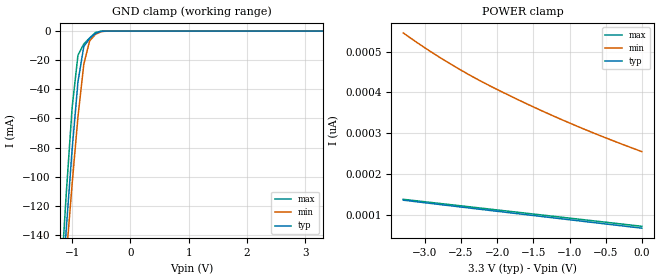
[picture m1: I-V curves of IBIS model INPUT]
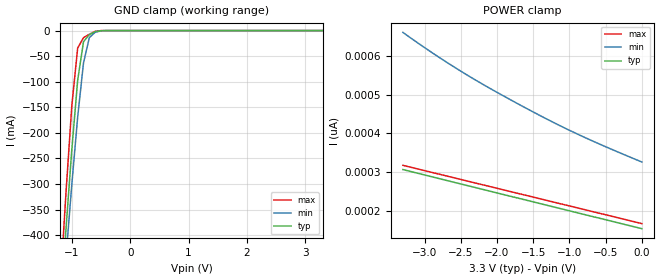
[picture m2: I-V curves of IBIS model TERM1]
|   PERICOM SEMICONDUCTOR CORP
|   IBIS Model of PI3C32X245
|   Product Family: 3C
|   BQSOP (B) Package
[IBIS Ver] 3.2
[Comment char] |_char
[File Name] pi3c32x245_b_33v.ibs
[File Rev] 2.0
[Source] File originated at Pericom Semiconductor Corp.
[Date] 03/15/18
[Disclaimer] (C) Copyright PERICOM Semiconductor Corporation
   All rights reserved
  Pericom Semiconductor Corporation hereby grants the user of
  this IBIS model a non-exclusive, nontransferable license to
  use this IBIS model under the following terms.
  This IBIS model is provided on an "AS IS" basis and Pericom
  makes absolutely no warranty with respect to the information
  contained herein. PERICOM DISCLAIMS AND CUSTOMER WAIVES ALL
  WARRANTIES, EXPRESSED OR IMPLIED, INCLUDING WARRANTIES OF
  MERCHANTABILITY OR FITNESS FOR A PARTICULAR PURPOSE. The
  entire risk as to quality and performance is with the customer.
  Accordingly, in no event shall the company be liable for any
  damages, whether in contract or tort, including any lost
  profits or other incidental, consequential, exemplary, or
  punitive damages arising out of the use or application of the
  IBIS model provided in this package. Further, Pericom reserves
  the right to make changes without notice to any product herein
  to improve reliability, function, or design. Pericom does not
  convey any license under patent rights or any other intellectual
  property rights, including those of third parties.
  The user is granted this license only to use the IBIS model
  and is not granted rights to sell, load, rent, lease or license
  the IBIS model in whole or in part, or in modified form to anyone
  other than user. User may modify the IBIS model to suit its specific
  application but rights to derivative works and such modifications
  shall belong to Pericom.
  Pericom is not obligated to provide maintenance or support
  for the licensed IBIS model.
  Contact Pericom at ATTN: APPLICATION ENGINEERING / IBIS MODELS
  2380 Bering Drive, San Jose, CA 95131
[Component] PI3C32X245
[Manufacturer] Pericom Semiconductor Corp.
[Package]
| Variable   typ   min   max
R_pkg   0.03818ohm   0.02666ohm   0.04970ohm
L_pkg   0.79246nH   0.73792nH   0.84700nH
C_pkg   0.19953pF   0.16164pF   0.23742pF
[Pin]  signal_name   model_name   R_pin   L_pin   C_pin
1   NC   NC   0.04970   0.84700nH   0.23742pF
2   A0   TERM1   0.04714   0.83488nH   0.22900pF
3   A1   TERM1   0.04458   0.82276nH   0.22058pF
4   A2   TERM1   0.04202   0.81064nH   0.21216pF
5   A3   TERM1   0.03946   0.79852nH   0.20374pF
6   A4   TERM1   0.03690   0.78640nH   0.19532pF
7   A5   TERM1   0.03434   0.77428nH   0.18690pF
8   A6   TERM1   0.03178   0.76216nH   0.17848pF
9   A7   TERM1   0.02922   0.75004nH   0.17006pF
10   GND   GND   0.02666   0.73792nH   0.16164pF
11   NC   NC   0.02666   0.73792nH   0.16164pF
12   A8   TERM1   0.02922   0.75004nH   0.17006pF
13   A9   TERM1   0.03178   0.76216nH   0.17848pF
14   A10   TERM1   0.03434   0.77428nH   0.18690pF
15   A11   TERM1   0.03690   0.78640nH   0.19532pF
16   A12   TERM1   0.03946   0.79852nH   0.20374pF
17   A13   TERM1   0.04202   0.81064nH   0.21216pF
18   A14   TERM1   0.04458   0.82276nH   0.22058pF
19   A15   TERM1   0.04714   0.83488nH   0.22900pF
20   GND   GND   0.04970   0.84700nH   0.23742pF
21   B15   TERM2   0.04970   0.84700nH   0.23742pF
22   B14   TERM2   0.04714   0.83488nH   0.22900pF
23   B13   TERM2   0.04458   0.82276nH   0.22058pF
24   B12   TERM2   0.04202   0.81064nH   0.21216pF
25   B11   TERM2   0.03946   0.79852nH   0.20374pF
26   B10   TERM2   0.03690   0.78640nH   0.19532pF
27   B9   TERM2   0.03434   0.77428nH   0.18690pF
28   B8   TERM2   0.03178   0.76216nH   0.17848pF
29   _BE2   INPUT   0.02922   0.75004nH   0.17006pF
30   VCC   POWER   0.02666   0.73792nH   0.16164pF
31   B7   TERM2   0.02666   0.73792nH   0.16164pF
32   B6   TERM2   0.02922   0.75004nH   0.17006pF
33   B5   TERM2   0.03178   0.76216nH   0.17848pF
34   B4   TERM2   0.03434   0.77428nH   0.18690pF
35   B3   TERM2   0.03690   0.78640nH   0.19532pF
36   B2   TERM2   0.03946   0.79852nH   0.20374pF
37   B1   TERM2   0.04202   0.81064nH   0.21216pF
38   B0   TERM2   0.04458   0.82276nH   0.22058pF
39   _BE1   INPUT   0.04714   0.83488nH   0.22900pF
40   VCC   POWER   0.04970   0.84700nH   0.23742pF
[Series Switch Groups]
On 1 /
Off 2 /
[Series Pin Mapping]   pin_2   model_name  function_table_group
2   38   SWITCH1   1
3   37   SWITCH1   1
4   36   SWITCH1   1
5   35   SWITCH1   1
6   34   SWITCH1   1
7   33   SWITCH1   1
8   32   SWITCH1   1
9   31   SWITCH1   1
12   28   SWITCH1   2
13   27   SWITCH1   2
14   26   SWITCH1   2
15   25   SWITCH1   2
16   24   SWITCH1   2
17   23   SWITCH1   2
18   22   SWITCH1   2
19   21   SWITCH1   2
|   Model SWITCH1
[Model] SWITCH1
Model_type Series_switch
| variable   typ   min   max
C_comp   10.000pF   9.800pF   10.200pF
[Voltage Range]   3.3000V   2.9700V   3.6300V
[GND Clamp Reference]   0.0000V   0.0000V   0.0000V
[POWER Clamp Reference]   3.3000V   2.9700V   3.6300V
[Temperature Range]   25   85   -40
[On]
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[OFF]
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| Models and submodels in the file (4): INPUT (Input), SWITCH1 (Series_switch), TERM1 (Terminator), TERM2 (Terminator)
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|   Model INPUT
[Model] INPUT
Model_type Input
Vinl = 800mV
Vinh = 2.0V
| variable   typ   min   max
C_comp   3.500pF   3.400pF   3.600pF
[Voltage Range]   3.3000V   2.9700V   3.6300V
[GND Clamp Reference]   0.0000V   0.0000V   0.0000V
[POWER Clamp Reference]   3.3000V   2.9700V   3.6300V
[Temperature Range]   25   85   -40
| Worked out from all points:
|   GND clamp passes 1 mA (typ) near -0.56 V on its own axis
[GND Clamp]
| Voltage   I(typ)   I(min)   I(max)
-3.3V     -1.504A    -1.38A     -1.677A
-1.2V     -193.5mA   -207.1mA   -176.6mA
-1.1V     -135.8mA   -155mA     -111.4mA
-1V       -81.33mA   -105mA     -52.61mA
-900mV    -34.92mA   -59.01mA   -16.58mA
-800mV    -10.56mA   -22.8mA    -8.882mA
-700mV    -5.104mA   -6.74mA    -4.717mA
-600mV    -1.611mA   -2.212mA   -981.9uA
-500mV    -145.9uA   -381.4uA   -24.42uA
-400mV    -4.329uA   -29.72uA   -133.6nA
3.3V      68.04pA    277.2pA    66pA
[POWER Clamp]   |Note: Vtable = Vcc - Voutput
| Voltage   I(typ)   I(min)   I(max)
-3.3V     136.5pA    545.5pA    138.6pA
-3V       130.2pA    509pA      132.6pA
-2.7V     123.9pA    475.3pA    126.6pA
-2.4V     117.6pA    444.3pA    120.6pA
-2V       109.3pA    407.1pA    112.6pA
-1.5V     98.92pA    364.5pA    102.6pA
-1V       88.6pA     325.2pA    92.6pA
-500mV    78.3pA     288.9pA    82.6pA
0V        68.04pA    255.2pA    72.6pA
|   Model TERM1
[Model] TERM1
Model_type Terminator
| variable   typ   min   max
C_comp   5.000pF   4.900pF   5.100pF
[Voltage Range]   3.3000V   2.9700V   3.6300V
[GND Clamp Reference]   0.0000V   0.0000V   0.0000V
[POWER Clamp Reference]   3.3000V   2.9700V   3.6300V
[Temperature Range]   25   85   -40
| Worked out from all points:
|   GND clamp passes 1 mA (typ) near -0.54 V on its own axis
[GND Clamp]
| Voltage   I(typ)   I(min)   I(max)
-3.3V     -4.264A    -3.909A    -4.763A
-1.2V     -551.9mA   -590.4mA   -503.2mA
-1.1V     -387.8mA   -442.8mA   -316.8mA
-1V       -232.2mA   -300.6mA   -146.4mA
-900mV    -97.23mA   -169.1mA   -34.28mA
-800mV    -21.65mA   -63.17mA   -13.78mA
-700mV    -7.82mA    -13.64mA   -7.205mA
-600mV    -2.298mA   -3.355mA   -1.407mA
-400mV    -5.736uA   -40.64uA   -175.6nA
3.3V      153pA      351.8pA    151pA
[POWER Clamp]   |Note: Vtable = Vcc - Voutput
| Voltage   I(typ)   I(min)   I(max)
-3.3V     306.2pA    661.9pA    317.2pA
-2.9V     287.5pA    609.6pA    298.9pA
-2.5V     268.9pA    561.3pA    280.6pA
-2.1V     250.3pA    516.9pA    262.3pA
-1.7V     231.7pA    475.6pA    244pA
-1.3V     213.2pA    436pA      225.6pA
-900mV    194.6pA    399.2pA    207.3pA
-500mV    176.1pA    365.5pA    189pA
0V        153pA      325.8pA    166.1pA
